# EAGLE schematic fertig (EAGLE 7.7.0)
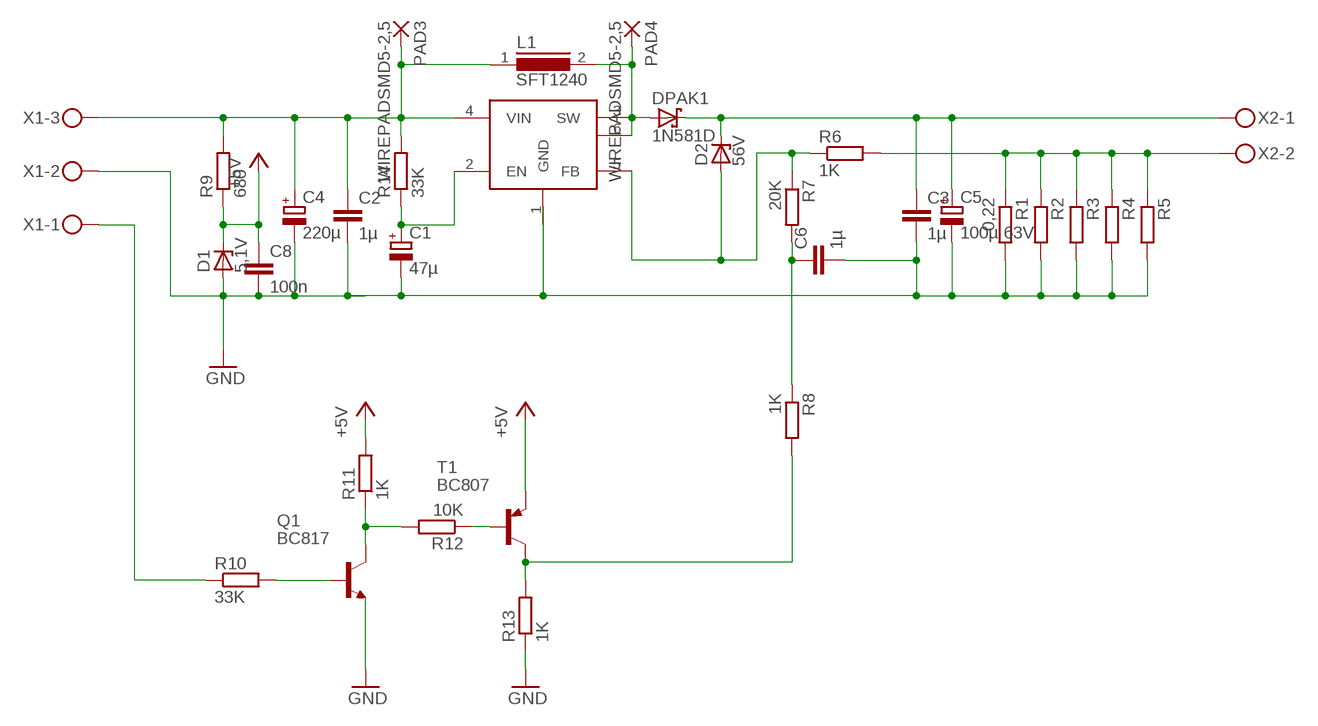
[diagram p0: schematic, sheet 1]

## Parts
C1  47µ  CPOL-EUE2.5-7  [E2,5-7]
C2  1µ  C-EUC1206K  [C1206K]
C3  1µ  C-EUC1206K  [C1206K]
C4  220µ  CPOL-EUE5-10.5  [E5-10,5]
C5  100µ 63V  CPOL-EUE5-10.5  [E5-10,5]
C6  1µ  C-EU050-075X075  [C050-075X075]
C8  100n  C-EUC1206  [C1206]
D1  5,1V  ZENER-DIODESOD80C  [SOD80C]
D2  56V  ZENER-DIODESOD80C  [SOD80C]
DPAK1  1N581D  [DPAK]
L1  SFT1240  [SFT1240]
PAD3  WIREPADSMD5-2,5  [5-2,5]
PAD4  WIREPADSMD5-2,5  [5-2,5]
Q1  BC817  BC817-16LT1SMD  [SOT23-BEC]
R1  0,22  R-EU_M1206  [M1206]
R2  R-EU_M1206  [M1206]
R3  R-EU_M1206  [M1206]
R4  R-EU_M1206  [M1206]
R5  R-EU_M1206  [M1206]
R6  1K  R-EU_M1206  [M1206]
R7  20K  R-EU_M1206  [M1206]
R8  1K  R-EU_M1206  [M1206]
R9  680  R-EU_R2512  [R2512]
R10  33K  R-EU_M1206  [M1206]
R11  1K  R-EU_M1206  [M1206]
R12  10K  R-EU_M1206  [M1206]
R13  1K  R-EU_M1206  [M1206]
R14  33K  R-EU_R1206  [R1206]
T1  BC807  BC807-16-PNP-SOT23-BEC  [SOT23-BEC]
U$1  XL6006  [TO263-5]
X1  MKDSN1,5/3-5,08  [MKDSN1,5/3-5,08]
X2  MKDSN1,5/2-5,08  [MKDSN1,5/2-5,08]

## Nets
+5V: C8.1 D1.C R9.1 R11.2 T1.E
N$1: C1.- C2.2 C3.2 C4.- C5.- C6.2 C8.2 D1.A Q1.E R1.2 R2.2 R3.2 R4.2 R5.2 R13.1 X1.2 ; supply symbol labelled GND
N$2: DPAK1.1(A) DPAK1.3(A) L1.2 PAD4.1(P) U$1.3(SW) U$1.6
N$3: C2.1 C4.+ L1.1 PAD3.1(P) R9.2 R14.2 U$1.4(VIN) X1.3
N$4: R1.1 R2.1 R3.1 R4.1 R5.1 R6.2 X2.2
N$5: C6.1 R7.2 R8.1
N$6: D2.A R6.1 R7.1 U$1.5(FB)
N$7: C3.1 C5.+ D2.C DPAK1.4(C) X2.1
N$8: Q1.C R11.1 R12.2
N$9: R12.1 T1.B
N$13: R8.2 R13.2 T1.C
N$14: Q1.B R10.2
N$15: R10.1 X1.1
N$134: C1.+ R14.1 U$1.2(EN)

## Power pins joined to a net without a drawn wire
GND: U$1.1(GND)

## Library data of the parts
C1 C4 C5 = rcl:CPOL-EU: POLARIZED CAPACITOR, European symbol
C2 C3 = resistor:C-EU: CAPACITOR, European symbol
C6 C8 = rcl:C-EU: CAPACITOR, European symbol
D1 D2 = diode:ZENER-DIODE: Z-Diode
DPAK1 = DPAK_Schottky:1N581*: 1.0A SCHOTTKY BARRIER RECTIFIER
L1 = inductors:SFT1240: INDUCTOR
PAD3 PAD4 = wirepad:WIREPAD: Wire PAD connect wire on PCB
Q1 = transistor-npn:BC817*: NPN Transistor
R1-R8 R10-R14 = rcl:R-EU_: RESISTOR, European symbol
R9 = resistor:R-EU_: RESISTOR, European symbol
T1 = transistor:*-PNP-: PNP Transistror
U$1 = XL6006:XL6006
X1 = con-phoenix-508:MKDSN1,5/3-5,08: MKDSN 1,5/ 3-5,08 Printklemme Nennstrom: 13,5 A Nennspannung: 250 V Rastermaß: 5,08 mm Polzahl: 3 Anschlussart: Schraubanschluss Montage: Löten Anschlussrichtung Leiter/Platine: 0 ° Artikelnummer: 1729131 Source: http://eshop.phoenixcontact.com .. 1729131.pdf
X2 = con-phoenix-508:MKDSN1,5/2-5,08: MKDSN 1,5/ 2-5,08 Printklemme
